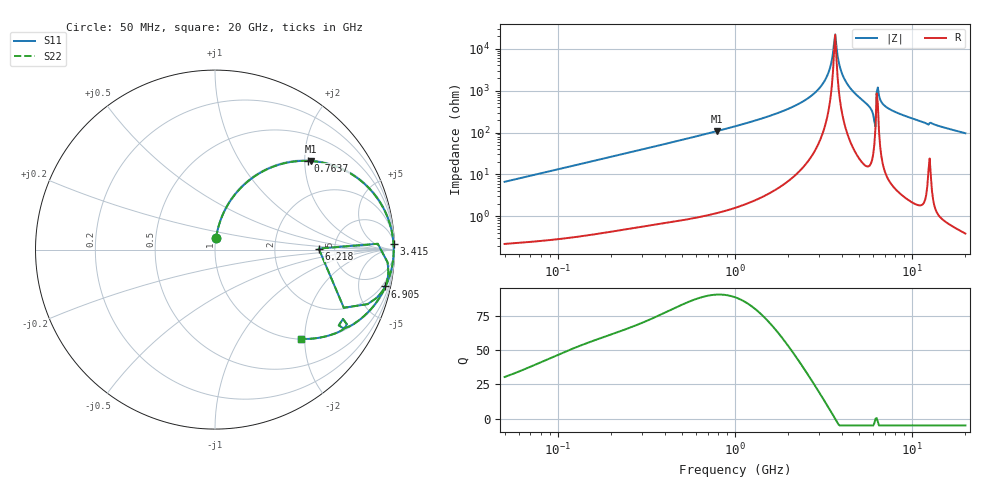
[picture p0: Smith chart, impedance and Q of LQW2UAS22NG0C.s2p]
!Murata Part Number: LQW2UAS22NG0C
!These Parameters are Measured in Series Mode Connection
!  o--[Z]--o
!Port1  Port2
!  o-------o
!Freq. Start=50[MHz] Stop=20[GHz], 401[Steps]
# Hz S RI R 50
!Freq.(Hz) S11(Real) S11(Imag) S21(Real) S21(Imag) S12(Real) S12(Imag) S22(Real) S22(Imag)
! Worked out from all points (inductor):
!   401 points, 50 MHz to 20 GHz, reference 50 ohm
!   read as one part in series: L = 21.1 nH near 51.52 MHz
!   highest Q = 90.8 at 786.9 MHz (marker M1), where L = 21.7 nH
!   self-resonance near 3.626 GHz
!   S11 on the Smith chart (normalised r, x): 50 MHz: 1.00, +0.13; 763.7 MHz: 1.02, +2.08; 3.415 GHz: 10, +63; 6.218 GHz: 3.74, +0.06; 6.905 GHz: 1.29, -9.18; 20 GHz: 1.01, -1.92
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5e7  0.00655 0.0659  0.9934 -0.0659  0.9934 -0.0659  0.00655 0.0659
1.364002e8  0.0344 0.1733  0.9656 -0.1733  0.9656 -0.1733  0.0344 0.1733
3.721004e8  0.1979 0.3919  0.8021 -0.3919  0.8021 -0.3919  0.1979 0.3919
7.636728e8  0.5195 0.4941  0.4805 -0.4941  0.4805 -0.4941  0.5195 0.4941
7.868965e8  0.5355 0.4933  0.4645 -0.4933  0.4645 -0.4933  0.5355 0.4933
1e9  0.6623 0.4673  0.3377 -0.4673  0.3377 -0.4673  0.6623 0.4673
1.848039e9  0.9075 0.2814  0.0925 -0.2814  0.0925 -0.2814  0.9075 0.2814
2.728004e9  0.9795 0.1245  0.0205 -0.1245  0.0205 -0.1245  0.9795 0.1245
3.121702e9  0.9907 0.0686  0.00929 -0.0686  0.00929 -0.0686  0.9907 0.0686
3.415248e9  0.9945 0.0309  0.00546 -0.0309  0.00546 -0.0309  0.9945 0.0309
3.572216e9  0.9954 0.012  0.00463 -0.012  0.00463 -0.012  0.9954 0.012
3.680849e9  0.9955 -0.000685  0.00448 0.000685  0.00448 0.000685  0.9955 -0.000685
3.967106e9  0.9944 -0.0327  0.00555 0.0327  0.00555 0.0327  0.9944 -0.0327
4.34015e9  0.9903 -0.0718  0.00973 0.0718  0.00973 0.0718  0.9903 -0.0718
5.683258e9  0.9423 -0.2159  0.0577 0.2159  0.0577 0.2159  0.9423 -0.2159
6.034176e9  0.8501 -0.3039  0.1499 0.3039  0.1499 0.3039  0.8501 -0.3039
6.217679e9  0.5779 0.00569  0.4221 -0.00569  0.4221 -0.00569  0.5779 0.00569
6.503449e9  0.9662 -0.1235  0.0338 0.1235  0.0338 0.1235  0.9662 -0.1235
6.905011e9  0.9488 -0.205  0.0512 0.205  0.0512 0.205  0.9488 -0.205
7.442007e9  0.9259 -0.2527  0.0741 0.2527  0.0741 0.2527  0.9259 -0.2527
1.183995e10  0.7399 -0.4315  0.2601 0.4315  0.2601 0.4315  0.7399 -0.4315
2e10  0.4809 -0.4976  0.5191 0.4976  0.5191 0.4976  0.4809 -0.4976
